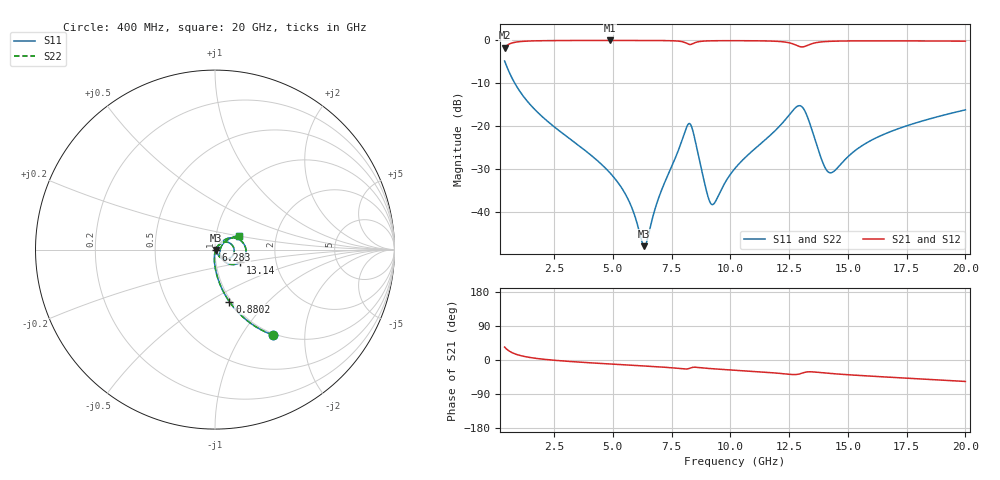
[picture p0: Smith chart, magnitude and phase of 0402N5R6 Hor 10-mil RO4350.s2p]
# GHz S MA R 50
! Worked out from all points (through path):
!   1960 points, 400 MHz to 20 GHz, reference 50 ohm
!   highest |S21| = -0.03 dB at 4.892 GHz (marker M1); lowest = -1.7 dB at 400 MHz (marker M2)
!   group delay of S21, straight-line fit = 9.08 ps
!   lowest |S11| = -48.0 dB at 6.343 GHz (marker M3), VSWR 1.01, Z = 50.4 - j0.142 ohm
!   |S11| at or under -10 dB: 833.4 MHz to end of sweep
!   |S22| runs from -48.0 to -4.8 dB; largest |S21 - S12| = 0
!   S11 on the Smith chart (normalised r, x): 400 MHz: 0.98, -1.39; 880.2 MHz: 0.98, -0.62; 6.283 GHz: 1.01, -0.01; 13.14 GHz: 1.31, -0.19; 20 GHz: 1.29, +0.20
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0.4  0.5744 -55.9  0.8183 34.1  0.8183 34.1  0.5744 -55.9
0.880245  0.3005 -74.6  0.953 15.3  0.953 15.3  0.3005 -74.6
1.860745  0.14 -86.0  0.9887 3.4  0.9887 3.4  0.14 -86.0
3.671669  0.05607 -93.7  0.996 -6.0  0.996 -6.0  0.05607 -93.7
4.892292  0.02833 -94.9  0.9966 -10.6  0.9966 -10.6  0.02833 -94.9
5.6927  0.01334 -89.1  0.9964 -13.4  0.9964 -13.4  0.01334 -89.1
6.283002  0.004193 -37.3  0.9958 -15.6  0.9958 -15.6  0.004193 -37.3
6.343032  0.003992 -20.6  0.9957 -15.8  0.9957 -15.8  0.003992 -20.6
6.943338  0.01434 50.0  0.9942 -18.0  0.9942 -18.0  0.01434 50.0
8.233997  0.1069 -1.1  0.8995 -22.7  0.8995 -22.7  0.1069 -1.1
8.404084  0.08888 -36.2  0.9142 -19.4  0.9142 -19.4  0.08888 -36.2
8.98438  0.01765 -46.6  0.9836 -21.8  0.9836 -21.8  0.01765 -46.6
9.194487  0.01231 -14.3  0.9874 -22.9  0.9874 -22.9  0.01231 -14.3
10.205  0.03232 48.2  0.9908 -27.0  0.9908 -27.0  0.03232 48.2
12.45615  0.1299 29.8  0.942 -37.4  0.942 -37.4  0.1299 29.8
12.87637  0.1717 1.4  0.8604 -37.8  0.8604 -37.8  0.1717 1.4
13.1365  0.1565 -27.2  0.8437 -33.1  0.8437 -33.1  0.1565 -27.2
13.46667  0.09149 -50.4  0.9126 -31.2  0.9126 -31.2  0.09149 -50.4
13.95692  0.03628 -38.5  0.9633 -33.9  0.9633 -33.9  0.03628 -38.5
14.25707  0.02858 -8.2  0.9739 -35.5  0.9739 -35.5  0.02858 -8.2
16.73834  0.08471 37.9  0.9857 -45.3  0.9857 -45.3  0.08471 37.9
20  0.1549 30.0  0.9779 -56.6  0.9779 -56.6  0.1549 30.0
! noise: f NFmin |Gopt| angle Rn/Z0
0.4  0.0008992  0.7154  3.311  0.0006235
2.571  0.005537  0.7017  6.778  0.003625
4.752  0.009431  0.6814  11.99  0.005671
6.933  0.01574  0.7174  17.2  0.01077
9.104  0.02851  0.7886  22.54  0.02672
11.29  0.02899  0.7506  27.63  0.02211
13.47  0.08957  0.897  32.94  0.1747
15.64  0.03488  0.7248  37.78  0.02259
17.82  0.03271  0.6797  42.43  0.01726
20  0.03431  0.6661  46.97  0.01671
